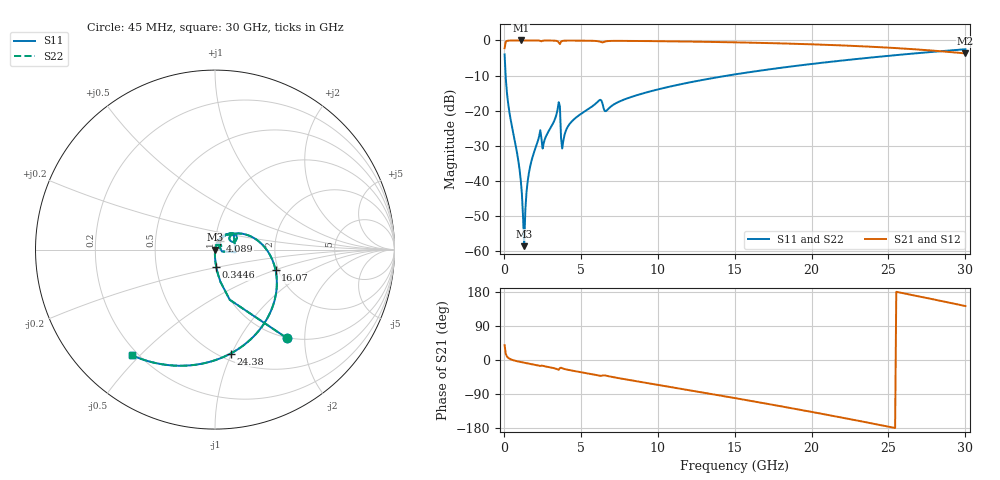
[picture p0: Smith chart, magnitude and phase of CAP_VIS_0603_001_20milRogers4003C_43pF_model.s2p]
! S-parameter model data by Modelithics Inc.  support@modelithics.com  813-866-6335  Tampa FL USA
! S-Parameter data specifications:
! Substrate: 20-mil Rogers 4003C, substrate thickness, H=0.508mm, Dielectric constant, Er=3.75
! PCB Mounting Pad Footprint: Pad width, PadW=0.90mm , Pad length, PadL=1.00mm , Pad gap, PadG (edge-to-edge)=1.00mm , Reference planes=3.0mm apart
! Created Wed Nov 18 13:28:50 2015
# hz S ma R 50
! 2 Port Network Data from SP1.SP block
! freq  magS11  angS11  magS21  angS21  magS12  angS12  magS22  angS22
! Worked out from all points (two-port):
!   401 points, 45 MHz to 30 GHz, reference 50 ohm
!   highest |S21| = -0.01 dB at 1.093 GHz (marker M1); lowest = -3.7 dB at 30 GHz (marker M2)
!   |S21| within 3 dB of the highest: start of sweep to 28.2 GHz
!   lowest |S11| = -58.6 dB at 1.318 GHz (marker M3), VSWR 1.00, Z = 50.1 + j0.0328 ohm
!   |S11| at or under -10 dB: 112 MHz to 14.55 GHz (14.44 GHz wide, 197 % of centre)
!   |S22| runs from -58.6 to -2.5 dB; largest |S21 - S12| = 0
!   S11 on the Smith chart (normalised r, x): 45 MHz: 0.99, -1.63; 344.6 MHz: 0.99, -0.20; 4.089 GHz: 1.05, +0.10; 16.07 GHz: 1.93, -0.50; 24.38 GHz: 0.56, -0.99; 30 GHz: 0.18, -0.47
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4.5e7  0.6328 -51.0  0.7742 39.0  0.7742 39.0  0.6328 -51.0
3.4455e8  0.09906 -85.8  0.9945 3.8  0.9945 3.8  0.09906 -85.8
8.687625e8  0.02391 -91.2  0.9988 -3.3  0.9988 -3.3  0.02391 -91.2
1.093425e9  0.01034 -89.9  0.9989 -5.3  0.9989 -5.3  0.01034 -89.9
1.168312e9  0.006557 -87.1  0.9989 -5.9  0.9989 -5.9  0.006557 -87.1
1.318088e9  0.001176 16.1  0.9988 -7.2  0.9988 -7.2  0.001176 16.1
1.692525e9  0.01554 75.3  0.9985 -10.0  0.9985 -10.0  0.01554 75.3
2.216738e9  0.03759 71.8  0.9964 -14.1  0.9964 -14.1  0.03759 71.8
2.666062e9  0.0395 68.9  0.9959 -16.7  0.9959 -16.7  0.0395 68.9
3.489825e9  0.1043 54.0  0.974 -24.7  0.974 -24.7  0.1043 54.0
3.864262e9  0.03743 51.9  0.9892 -22.9  0.9892 -22.9  0.03743 51.9
4.088925e9  0.05573 60.2  0.9937 -25.3  0.9937 -25.3  0.05573 60.2
5.062462e9  0.09161 55.6  0.9925 -32.6  0.9925 -32.6  0.09161 55.6
6.185775e9  0.1395 39.7  0.9681 -41.3  0.9681 -41.3  0.1395 39.7
6.709988e9  0.1018 38.2  0.977 -41.9  0.977 -41.9  0.1018 38.2
1.007992e10  0.2023 23.1  0.9752 -66.0  0.9752 -66.0  0.2023 23.1
1.50225e10  0.3284 -11.2  0.9394 -100.5  0.9394 -100.5  0.3284 -11.2
1.607092e10  0.356 -18.7  0.9291 -108.0  0.9291 -108.0  0.356 -18.7
2.003996e10  0.4631 -47.8  0.8798 -137.2  0.8798 -137.2  0.4631 -47.8
2.438344e10  0.5857 -81.5  0.8024 -171.0  0.8024 -171.0  0.5857 -81.5
2.505742e10  0.6052 -86.9  0.7877 -176.4  0.7877 -176.4  0.6052 -86.9
3e10  0.7484 -128.1  0.6523 142.4  0.6523 142.4  0.7484 -128.1
